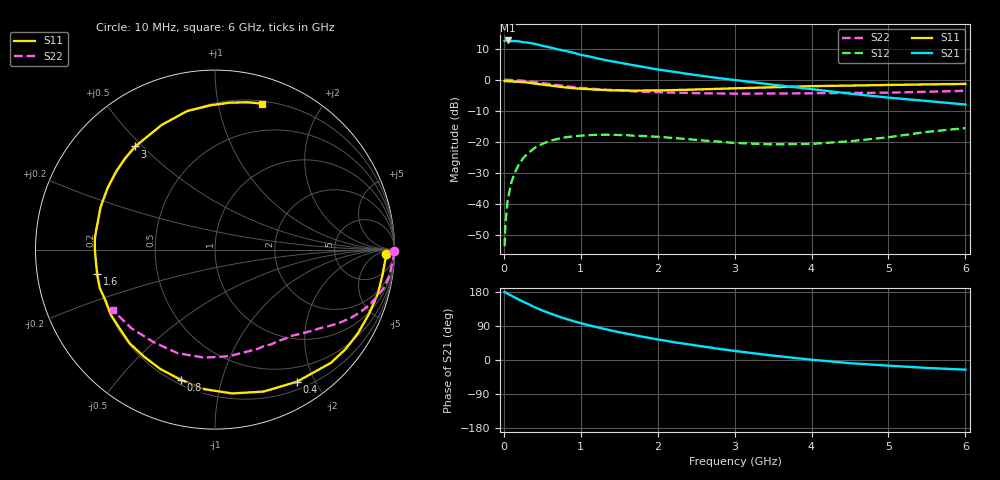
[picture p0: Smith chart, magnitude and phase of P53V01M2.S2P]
! SIEMENS Small Signal Semiconductors
! BFP183
! Si NPN RF Bipolar Junction Transistor in SOT143
! VCE = 3 V  IC = 1.2 mA
! Common Emitter S-Parameters:  March  1996
# GHz  S  MA  R  50
!  f  S11  S21  S12  S22
! GHz  MAG  ANG  MAG  ANG  MAG  ANG  MAG  ANG
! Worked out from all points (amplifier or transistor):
!   36 points, 10 MHz to 6 GHz, reference 50 ohm
!   highest |S21| = 12.6 dB at 50 MHz (marker M1)
!   |S21| within 3 dB of that: start of sweep to 728.6 MHz
!   unconditionally stable (mu >= 1): 2.401 GHz to end of sweep
!   at 250 MHz: K = 0.10, MSG = 18.7 dB, |S12| = -25.3 dB
!   at 1.4 GHz: K = 0.56, MSG = 11.8 dB, |S12| = -17.7 dB
!   at 6 GHz: K = 1.02, MAG = 3.0 dB, |S12| = -15.6 dB
!   S11 on the Smith chart (normalised r, x): 10 MHz: 33, -17; 400 MHz: 0.30, -1.76; 800 MHz: 0.23, -0.75; 1.6 GHz: 0.20, -0.10; 3 GHz: 0.20, +0.48; 6 GHz: 0.22, +1.35
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0.01  0.9532 -1.4  4.211 179.3  0.0021 90.1  0.9998 -0.5
0.02  0.9513 -3.1  4.27 178.6  0.0047 85.7  0.9993 -1.1
0.05  0.9443 -7.9  4.279 174.7  0.0115 86.5  0.995 -2.6
0.1  0.9405 -14.9  4.16 169.6  0.0229 80.7  0.9873 -5.3
0.15  0.9296 -22.9  4.18 164.1  0.0335 76.5  0.9839 -8.1
0.2  0.9229 -30.3  4.133 158.9  0.0442 72.7  0.9742 -10.6
0.3  0.9028 -44.3  3.964 149.4  0.0634 64.0  0.9462 -15.3
0.4  0.8661 -58.2  3.789 139.3  0.0797 56.0  0.9153 -19.6
0.5  0.836 -71.1  3.513 130.7  0.0927 49.0  0.8801 -23.4
0.6  0.8072 -83.2  3.307 123.0  0.104 42.7  0.8489 -26.5
0.8  0.7504 -104.5  2.911 109.0  0.1183 32.2  0.7898 -31.7
0.9  0.7318 -114.6  2.721 102.9  0.1231 27.7  0.7628 -34.0
1.1  0.7065 -132.2  2.379 91.7  0.1281 20.3  0.7225 -37.7
1.4  0.673 -154.9  1.981 77.7  0.1299 11.3  0.6822 -42.8
1.6  0.6706 -168.3  1.787 69.4  0.1282 7.0  0.6607 -45.7
1.8  0.6696 179.6  1.614 61.5  0.1245 3.9  0.6393 -48.9
2.2  0.6804 159.4  1.348 47.4  0.1155 -0.8  0.6183 -55.7
3  0.7267 127.7  0.99 23.9  0.0961 -0.5  0.5964 -71.5
3.5  0.7555 113.1  0.83 11.5  0.091 6.0  0.599 -82.5
4.5  0.8046 91.7  0.597 -8.4  0.1024 21.1  0.6136 -109.9
5.5  0.84 77.7  0.454 -20.9  0.1447 26.0  0.6396 -136.7
6  0.8556 72.0  0.399 -25.5  0.1665 23.0  0.6624 -149.4
